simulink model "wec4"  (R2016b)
settings: Solver=ode4  StartTime=0  StopTime=1000  FixedStep=0.005  MaxStep=0.005  RelTol=1e-3  EnableMultiTasking=on
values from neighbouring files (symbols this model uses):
  arAdaptiveLawData = 1/2*zModelSimple.zModelPto.arFreq.*     zModelSimple.zModelPto.arMagnitude./     cos(zModelSimple.zModelPto.arPhase*pi/180+pi/2)    [IMPACT_Control.m]
  arAdaptiveLawDataX = 1/2*zModelSimpleX.zModelPto.arFreq.*         zModelSimpleX.zModelPto.arMagnitude./         cos(zModelSimpleX.zModelPto.arPhase*pi/180+pi/2)    [IMPACT_Control.m]
  arControllerRampGain = [0,0,1,1]    [IMPACT_Control.m]
  arControllerRampTime = [0 rStartRampTime rStartRampTime+rRampTimeLength 8000]    [IMPACT_Control.m]
  arEkfInitialisation = zeros(1,11)    [IMPACT_Control.m]
  arEkfInitialisationX = zeros(1,11)    [IMPACT_Control.m]
  arFrequency = zModelSimple.zModelPto.arFreq    [IMPACT_Control.m]
  arFrequencyRange = zModelSimple.zModelPto.arFreq    [IMPACT_Control.m]
  arFrequencyX = zModelSimpleX.zModelPto.arFreq    [IMPACT_Control.m]
  arImpedance = 1./zModelSimple.zModelPto.arMagnitude./zModelSimple.zModelPto.arFreq    [IMPACT_Control.m]
  arImpedanceX = 1./zModelSimpleX.zModelPto.arMagnitude./zModelSimpleX.zModelPto.arFreq    [IMPACT_Control.m]
  CentralPTOPreload = -1.6113e+07    (= -16113000)    [wecSimInputFile.m]
  F1 = [4.243 2.375 -12.243]    [wecSimInputFile.m]
  F2 = [4.243 -2.375 -12.243]    [wecSimInputFile.m]
  F3 = [-4.243 -2.375 -12.243]    [wecSimInputFile.m]
  F4 = [-4.243 2.375 -12.243]    [wecSimInputFile.m]
  FC = [0 0 -14]    [wecSimInputFile.m]
  iAdaptiveDamping = 0    [wec4IMPACT_Project.m]    (also in IMPACT_Control.m = handles.iAdaptiveDamping; wec1_IMPACT_Project.m; wec2_IMPACT_Project.m; wec3_IMPACT_Project.m)
  iControlType = 2    [wec4IMPACT_Project.m]    (also in IMPACT_Control.m = handles.iControlType; wec1_IMPACT_Project.m = 1; wec2_IMPACT_Project.m = 1; wec3_IMPACT_Project.m = 1)
  iPtoPositionConstraint = 1    [wec4IMPACT_Project.m]    (also in IMPACT_Control.m = handles.iPtoPositionConstraint; wec1_IMPACT_Project.m = 0; wec2_IMPACT_Project.m; wec3_IMPACT_Project.m)
  iSensorNoise = 0    [IMPACT_Control.m]
  m = m+1    (= 2)    [checkParamFile.m]
  PTOrotation = atan((T1(2)-F1(2))/(T1(1)-F1(1)))    [wecSimInputFile.m]
  rCogFloater = -8    [wec4_IMPACT_Model.m]    (also in paramInitial.m = get( handles.edit_rCogFloater, 'String' ); wec1_IMPACT_Model.m = -18; wec2_IMPACT_Model.m = -8.5; wec3_IMPACT_Model.m = -0.7)
  rCogSpar = -36.6    [wec4_IMPACT_Model.m]    (also in paramInitial.m = get( handles.edit_rCogSpar, 'String' ); wec3_IMPACT_Model.m = -21.3; wec3_IMPACT_Model2.m = -21.3)
  rDisplacementLimit = 10.000000    (= 10)    [wec4IMPACT_Project.m]    (also in IMPACT_Control.m = getValue(handles.edit_displacementLimit); wec1_IMPACT_Project.m; wec2_IMPACT_Project.m; wec3_IMPACT_Project.m = 3)
  rDisplacementLimitX = 10.000000    (= 10)    [wec4IMPACT_Project.m]    (also in IMPACT_Control.m = getValue(handles.edit_displacementLimitX); wec1_IMPACT_Project.m = 0; wec2_IMPACT_Project.m; wec3_IMPACT_Project.m = 0)
  rGainForAntiWIndUp = tfControllerDiscrete.rGain    [IMPACT_Control.m]
  rGainForAntiWIndUpX = tfControllerXDiscrete.rGain    [IMPACT_Control.m]
  rMaxForcePto = 300000000.000000    (= 300000000)    [wec4IMPACT_Project.m]    (also in IMPACT_Control.m = getValue(handles.edit_maxForcePto); wec1_IMPACT_Project.m = 1e+15; wec2_IMPACT_Project.m = 1e+15; wec3_IMPACT_Project.m = 1000000000)
  rMinForcePto = -300000000.000000    (= -300000000)    [wec4IMPACT_Project.m]    (also in IMPACT_Control.m = getValue(handles.edit_minForcePto); wec1_IMPACT_Project.m = -1e+15; wec2_IMPACT_Project.m = -1e+15; wec3_IMPACT_Project.m = -1000000000)
  rMooringX = 20000    [wec4_IMPACT_Model.m]    (also in paramInitial.m = get( handles.edit_rMooringX, 'String' ); wec3_IMPACT_Model.m = 10000; wec3_IMPACT_Model2.m = 10000)
  rMooringZ = 10000    [wec4_IMPACT_Model.m]    (also in paramInitial.m = get( handles.edit_rMooringZ, 'String' ); wec3_IMPACT_Model.m = 0; wec3_IMPACT_Model2.m = 0)
  rOutputSampleTime = 0.010000    (= 0.01)    [wec4IMPACT_Project.m]    (also in IMPACT_Control.m = getValue(handles.edit_outputSampleTime); wec1_IMPACT_Project.m; wec2_IMPACT_Project.m; wec3_IMPACT_Project.m)
  rPassiveDampingGain = -604830.000000    (= -604830)    [wec4IMPACT_Project.m]    (also in IMPACT_Control.m = getValue(handles.edit_gainPLD); wec1_IMPACT_Project.m = -214018.1537; wec2_IMPACT_Project.m = -1948070; wec3_IMPACT_Project.m = -519390)
  rPassiveDampingGainX = -278660.000000    (= -278660)    [wec4IMPACT_Project.m]    (also in IMPACT_Control.m = getValue(handles.edit_gainPLDX); wec1_IMPACT_Project.m = 0; wec2_IMPACT_Project.m = 0; wec3_IMPACT_Project.m = 0)
  rTetherPretension = 1.6113e+07    (= 16113000)    [wec4_IMPACT_Model.m]    (also in paramInitial.m = get( handles.edit_rTetherPretension, 'String' ); wec3_IMPACT_Model.m = 0; wec3_IMPACT_Model2.m = 0)
  rTetherSpring = 500000    [wec4_IMPACT_Model.m]    (also in paramInitial.m = get( handles.edit_rTetherSpring, 'String' ); wec3_IMPACT_Model.m = 0; wec3_IMPACT_Model2.m = 0)
  rUpperFrequencyLimit = EKFFloater.upperFreq    [IMPACT_Control.m]
  rXf = 4.243    [wec4AdditionalParams.m]
  rXs = 16.075    [wec4AdditionalParams.m]
  rYf = 2.375    [wec4AdditionalParams.m]
  rYs = 16.075    [wec4AdditionalParams.m]
  rZf = 4.243    [wec4AdditionalParams.m]
  rZs = 2.4350    (= 2.435)    [wec4AdditionalParams.m]
  rZTetherF = 6    [wec4AdditionalParams.m]
  rZTetherS = 2.4350    (= 2.435)    [wec4AdditionalParams.m]
  s = tf('s')    [wec4_IMPACT_Model.m]    (also in IMPACT_Control.m; wec1_IMPACT_Model.m; wec2_IMPACT_Model.m; wec3_IMPACT_Model.m)
  SidePTO1Preload = PreloadPTOCorner    (= 0)    [wecSimInputFile.m]
  SidePTO2Preload = PreloadPTOCorner    (= 0)    [wecSimInputFile.m]
  SidePTO3Preload = PreloadPTOCorner    (= 0)    [wecSimInputFile.m]
  SidePTO4Preload = PreloadPTOCorner    (= 0)    [wecSimInputFile.m]
  simu = simulationClass()    [wecSimInputFile.m]
  T1 = [16.075 16.075 -34.165]    [wecSimInputFile.m]
  T2 = [16.075 -16.075 -34.165]    [wecSimInputFile.m]
  T3 = [-16.075 -16.075 -34.165]    [wecSimInputFile.m]
  T4 = [-16.075 16.075 -34.165]    [wecSimInputFile.m]
  TC = [0 0 -34.165]    [wecSimInputFile.m]
  waves = waveClass('irregular')    [wecSimInputFile.m]
  Z = magPhaseToComplex(zModelTf)    [IMPACT_Control.m]
undefined symbols (not defined in the file or in its folder): arControllerDiscreteDen, arControllerDiscreteNum, arControllerDiscreteXDen, arControllerDiscreteXNum, arExcForceFloaterDen, arExcForceFloaterNum, arExcForceFloaterXDen, arExcForceFloaterXNum, arExcForceSparDen, arExcForceSparNum, arExcForceSparXDen, arExcForceSparXNum, arFexcFloaterDen, arFexcFloaterNum, arFexcFloaterXDen, arFexcFloaterXNum, arFexcSparDen, arFexcSparNum, arFexcSparXDen, arFexcSparXNum, Body, body, constraint, CTTime, deg, Elements, geometry, IRKB, kg, lenJ, mooring, N, pto, rAccelerationGainFloater, rAccelerationGainFloaterX, rAccelerationGainSpar, rAccelerationGainSparX, rad, rBuoyancyGainFloater, rBuoyancyGainFloaterX, rBuoyancyGainSpar, rBuoyancyGainSparX, rDampingGainFloater, rDampingGainFloaterX, rDampingGainSpar, rDampingGainSparX, Rigid, rMaxFocePto, wec4_float, wec4_reactor, WECSim_Lib, X, Y
libraries: nesl_utility x380, sm_lib x170, vrlib x91, simulink x12, WECSim_Lib x4
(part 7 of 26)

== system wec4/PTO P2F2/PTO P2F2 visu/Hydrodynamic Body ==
  Additional Linear Damping Force Calculation : Subsystem
  B2B Subsystem : Subsystem  Variant=on
  Bus Creator : BusCreator  Inputs=6
  Bus Creator1 : BusCreator  Inputs=3
  Bus Selector1 : BusSelector  OutputSignals=F_Excitation,F_RadiationDamping,F_AddedMass,F_Restoring,F_MorrisonAndViscous,F_LinearDamping
  Bus Selector2 : BusSelector  OutputSignals=disp,vel,acc
  Hydrostatic Restoring Force Calculation : Subsystem
  Morrison Element and ViscousDampingForceCalculation : Subsystem
  Nonlinear Wave Elevation : Subsystem  TreatAsAtomicUnit=on  SystemSampleTime=simu.dtNL
  Structure : Subsystem
  Sum : Sum  Inputs=+-----
  To Workspace : ToWorkspace  VariableName=body5_out  SaveFormat=Structure With Time  SampleTime=-1
  Wave Diffraction and Excitation Force Calculation : Subsystem
  Wave Radiation Forces Calculation : Subsystem
  Conn : PMIOPort  Port=1  Side=Right
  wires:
  Additional Linear Damping Force Calculation/1(F_LinearDamping) -> Bus Creator/6
  Bus Creator/1 -> Bus Selector1/1, Bus Creator1/3  "BUS(7): Forces"
  Bus Selector2/1 -> [disp5]  "<disp>"
  Bus Selector2/3 -> [acc5]  "<acc>"
  Bus Selector2/2 -> [vel5]  "<vel>"
  Structure/1(Response) -> Bus Creator1/1, Bus Selector2/1
  Sum/1 -> Bus Creator1/2, Structure/1(Total Force)  "F_Total"
  Bus Creator1/1 -> To Workspace/1
  Bus Selector1/4 -> Sum/4  "<F_Restoring>"
  Bus Selector1/3 -> Sum/3  "<F_AddedMass>"
  Bus Selector1/5 -> Sum/5  "<F_MorrisonAndViscous>"
  Bus Selector1/2 -> Sum/2  "<F_RadiationDamping>"
  Bus Selector1/1 -> Sum/1  "<F_Excitation>"
  Bus Selector1/6 -> Sum/6  "<F_LinearDamping>"
  [acc5] -> B2B Subsystem/2(acc_in), Morrison Element and ViscousDampingForceCalculation/2(Acceleration)
  [vel5] -> Morrison Element and ViscousDampingForceCalculation/3(Velocity), Additional Linear Damping Force Calculation/1(Velocity), B2B Subsystem/1(vel_in)
  B2B Subsystem/2(acc) -> Wave Radiation Forces Calculation/2(Acceleration)
  B2B Subsystem/1(vel) -> Wave Radiation Forces Calculation/1(Velocity)
  [disp5] -> Hydrostatic Restoring Force Calculation/1(Displacement), Morrison Element and ViscousDampingForceCalculation/1(Displacement), Nonlinear Wave Elevation/1(Displacement), Wave Diffraction and Excitation Force Calculation/2(Displacement)
  Nonlinear Wave Elevation/1(Wave Elevation) -> Wave Diffraction and Excitation Force Calculation/3(WaveElv), Hydrostatic Restoring Force Calculation/2(Wave Elv)
  Hydrostatic Restoring Force Calculation/1(F_Restoring) -> Bus Creator/4
  Wave Radiation Forces Calculation/1(F_RadiationDamping) -> Bus Creator/2
  Wave Diffraction and Excitation Force Calculation/1(F_Excitation) -> Bus Creator/1
  Wave Radiation Forces Calculation/2(F_AddedMass) -> Bus Creator/3
  [Clock] -> Nonlinear Wave Elevation/2(Time), Wave Diffraction and Excitation Force Calculation/1(Time), Morrison Element and ViscousDampingForceCalculation/4(Time), Wave Radiation Forces Calculation/3(Time)
  Morrison Element and ViscousDampingForceCalculation/1(F_MorrisonAndViscous) -> Bus Creator/5
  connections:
  Conn/RConn1 -- Structure/RConn1

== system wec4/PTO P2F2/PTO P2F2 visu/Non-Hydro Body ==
  Bus Creator : BusCreator  Inputs=6
  Bus Creator1 : BusCreator  Inputs=3
  Bus Selector1 : BusSelector  OutputSignals=F_Excitation,F_RadiationDamping,F_AddedMass,F_Restoring,F_MorrisonAndViscous,F_LinearDamping
  Constant{,1..3,5} (5 alike) : Constant  Value=[0 0 0 0 0 0]
  Structure : Subsystem
  Sum : Sum  Inputs=+-----
  To Workspace : ToWorkspace  VariableName=body5_out  SaveFormat=Structure With Time  SampleTime=-1
  Weight and Buoyancy : Subsystem
  Conn : PMIOPort  Port=1  Side=Right
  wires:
  Bus Creator/1 -> Bus Creator1/3, Bus Selector1/1  "BUS(7): Forces"
  Structure/1(Response) -> Bus Creator1/1
  Sum/1 -> Bus Creator1/2, Structure/1(Total Force)  "F_Total"
  Bus Creator1/1 -> To Workspace/1
  Bus Selector1/4 -> Sum/4  "<F_Restoring>"
  Bus Selector1/3 -> Sum/3  "<F_AddedMass>"
  Bus Selector1/5 -> Sum/5  "<F_MorrisonAndViscous>"
  Bus Selector1/2 -> Sum/2  "<F_RadiationDamping>"
  Bus Selector1/1 -> Sum/1  "<F_Excitation>"
  Bus Selector1/6 -> Sum/6  "<F_LinearDamping>"
  Constant5/1 -> Bus Creator/6  "F_LinearDamping"
  Constant3/1 -> Bus Creator/5  "F_MorrisonAndViscous"
  Constant2/1 -> Bus Creator/3  "F_AddedMass"
  Constant1/1 -> Bus Creator/2  "F_RadiationDamping"
  Constant/1 -> Bus Creator/1  "F_Excitation"
  Weight and Buoyancy/1(Out1) -> Bus Creator/4  "F_Restoring"
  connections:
  Conn/RConn1 -- Structure/RConn1

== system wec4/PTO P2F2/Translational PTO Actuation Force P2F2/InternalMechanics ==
  note: Calculate PTO force and power. F_pto = k*x + c*v, where F_pto is the force the PTO applies to the body (at the PTO location), x and v are the joint position and velocity. The power extracted is P = c * v^2
  Position : Inport
  Velocity : Inport  Port=2
  Add : Sum  Inputs=--
  Math Function : Math  Operator=square
  PCC Damping Coefficient : Constant  Value=pto.c
  PCC Stiffness Coefficient : Constant  Value=pto.k
  Product : Product  Inputs=**
  Product1 : Product  Inputs=**
  Product2 : Product  Inputs=**
  Force : Outport
  Power : Outport  Port=2
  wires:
  PCC Damping Coefficient/1 -> Product2/1, Product1/1
  Product2/1 -> Power/1
  Velocity/1 -> Math Function/1, Product1/2
  PCC Stiffness Coefficient/1 -> Product/2
  Position/1 -> Product/1
  Add/1 -> Force/1
  Math Function/1 -> Product2/2
  Product/1 -> Add/1
  Product1/1 -> Add/2

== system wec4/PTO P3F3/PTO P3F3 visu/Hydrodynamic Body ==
  Additional Linear Damping Force Calculation : Subsystem
  B2B Subsystem : Subsystem  Variant=on
  Bus Creator : BusCreator  Inputs=6
  Bus Creator1 : BusCreator  Inputs=3
  Bus Selector1 : BusSelector  OutputSignals=F_Excitation,F_RadiationDamping,F_AddedMass,F_Restoring,F_MorrisonAndViscous,F_LinearDamping
  Bus Selector2 : BusSelector  OutputSignals=disp,vel,acc
  Hydrostatic Restoring Force Calculation : Subsystem
  Morrison Element and ViscousDampingForceCalculation : Subsystem
  Nonlinear Wave Elevation : Subsystem  TreatAsAtomicUnit=on  SystemSampleTime=simu.dtNL
  Structure : Subsystem
  Sum : Sum  Inputs=+-----
  To Workspace : ToWorkspace  VariableName=body6_out  SaveFormat=Structure With Time  SampleTime=-1
  Wave Diffraction and Excitation Force Calculation : Subsystem
  Wave Radiation Forces Calculation : Subsystem
  Conn : PMIOPort  Port=1  Side=Right
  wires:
  Additional Linear Damping Force Calculation/1(F_LinearDamping) -> Bus Creator/6
  Bus Creator/1 -> Bus Selector1/1, Bus Creator1/3  "BUS(7): Forces"
  Bus Selector2/1 -> [disp6]  "<disp>"
  Bus Selector2/3 -> [acc6]  "<acc>"
  Bus Selector2/2 -> [vel6]  "<vel>"
  Structure/1(Response) -> Bus Creator1/1, Bus Selector2/1
  Sum/1 -> Bus Creator1/2, Structure/1(Total Force)  "F_Total"
  Bus Creator1/1 -> To Workspace/1
  Bus Selector1/4 -> Sum/4  "<F_Restoring>"
  Bus Selector1/3 -> Sum/3  "<F_AddedMass>"
  Bus Selector1/5 -> Sum/5  "<F_MorrisonAndViscous>"
  Bus Selector1/2 -> Sum/2  "<F_RadiationDamping>"
  Bus Selector1/1 -> Sum/1  "<F_Excitation>"
  Bus Selector1/6 -> Sum/6  "<F_LinearDamping>"
  [acc6] -> B2B Subsystem/2(acc_in), Morrison Element and ViscousDampingForceCalculation/2(Acceleration)
  [vel6] -> Morrison Element and ViscousDampingForceCalculation/3(Velocity), Additional Linear Damping Force Calculation/1(Velocity), B2B Subsystem/1(vel_in)
  B2B Subsystem/2(acc) -> Wave Radiation Forces Calculation/2(Acceleration)
  B2B Subsystem/1(vel) -> Wave Radiation Forces Calculation/1(Velocity)
  [disp6] -> Hydrostatic Restoring Force Calculation/1(Displacement), Morrison Element and ViscousDampingForceCalculation/1(Displacement), Nonlinear Wave Elevation/1(Displacement), Wave Diffraction and Excitation Force Calculation/2(Displacement)
  Nonlinear Wave Elevation/1(Wave Elevation) -> Wave Diffraction and Excitation Force Calculation/3(WaveElv), Hydrostatic Restoring Force Calculation/2(Wave Elv)
  Hydrostatic Restoring Force Calculation/1(F_Restoring) -> Bus Creator/4
  Wave Radiation Forces Calculation/1(F_RadiationDamping) -> Bus Creator/2
  Wave Diffraction and Excitation Force Calculation/1(F_Excitation) -> Bus Creator/1
  Wave Radiation Forces Calculation/2(F_AddedMass) -> Bus Creator/3
  [Clock] -> Nonlinear Wave Elevation/2(Time), Wave Diffraction and Excitation Force Calculation/1(Time), Morrison Element and ViscousDampingForceCalculation/4(Time), Wave Radiation Forces Calculation/3(Time)
  Morrison Element and ViscousDampingForceCalculation/1(F_MorrisonAndViscous) -> Bus Creator/5
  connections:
  Conn/RConn1 -- Structure/RConn1

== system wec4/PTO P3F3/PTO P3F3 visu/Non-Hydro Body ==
  Bus Creator : BusCreator  Inputs=6
  Bus Creator1 : BusCreator  Inputs=3
  Bus Selector1 : BusSelector  OutputSignals=F_Excitation,F_RadiationDamping,F_AddedMass,F_Restoring,F_MorrisonAndViscous,F_LinearDamping
  Constant{,1..3,5} (5 alike) : Constant  Value=[0 0 0 0 0 0]
  Structure : Subsystem
  Sum : Sum  Inputs=+-----
  To Workspace : ToWorkspace  VariableName=body6_out  SaveFormat=Structure With Time  SampleTime=-1
  Weight and Buoyancy : Subsystem
  Conn : PMIOPort  Port=1  Side=Right
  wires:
  Bus Creator/1 -> Bus Creator1/3, Bus Selector1/1  "BUS(7): Forces"
  Structure/1(Response) -> Bus Creator1/1
  Sum/1 -> Bus Creator1/2, Structure/1(Total Force)  "F_Total"
  Bus Creator1/1 -> To Workspace/1
  Bus Selector1/4 -> Sum/4  "<F_Restoring>"
  Bus Selector1/3 -> Sum/3  "<F_AddedMass>"
  Bus Selector1/5 -> Sum/5  "<F_MorrisonAndViscous>"
  Bus Selector1/2 -> Sum/2  "<F_RadiationDamping>"
  Bus Selector1/1 -> Sum/1  "<F_Excitation>"
  Bus Selector1/6 -> Sum/6  "<F_LinearDamping>"
  Constant5/1 -> Bus Creator/6  "F_LinearDamping"
  Constant3/1 -> Bus Creator/5  "F_MorrisonAndViscous"
  Constant2/1 -> Bus Creator/3  "F_AddedMass"
  Constant1/1 -> Bus Creator/2  "F_RadiationDamping"
  Constant/1 -> Bus Creator/1  "F_Excitation"
  Weight and Buoyancy/1(Out1) -> Bus Creator/4  "F_Restoring"
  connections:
  Conn/RConn1 -- Structure/RConn1

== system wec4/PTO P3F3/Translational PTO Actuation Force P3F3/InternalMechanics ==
  note: Calculate PTO force and power. F_pto = k*x + c*v, where F_pto is the force the PTO applies to the body (at the PTO location), x and v are the joint position and velocity. The power extracted is P = c * v^2
  Position : Inport
  Velocity : Inport  Port=2
  Add : Sum  Inputs=--
  Math Function : Math  Operator=square
  PCC Damping Coefficient : Constant  Value=pto.c
  PCC Stiffness Coefficient : Constant  Value=pto.k
  Product : Product  Inputs=**
  Product1 : Product  Inputs=**
  Product2 : Product  Inputs=**
  Force : Outport
  Power : Outport  Port=2
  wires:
  PCC Damping Coefficient/1 -> Product2/1, Product1/1
  Product2/1 -> Power/1
  Velocity/1 -> Math Function/1, Product1/2
  PCC Stiffness Coefficient/1 -> Product/2
  Position/1 -> Product/1
  Add/1 -> Force/1
  Math Function/1 -> Product2/2
  Product/1 -> Add/1
  Product1/1 -> Add/2

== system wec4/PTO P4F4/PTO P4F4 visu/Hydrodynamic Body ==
  Additional Linear Damping Force Calculation : Subsystem
  B2B Subsystem : Subsystem  Variant=on
  Bus Creator : BusCreator  Inputs=6
  Bus Creator1 : BusCreator  Inputs=3
  Bus Selector1 : BusSelector  OutputSignals=F_Excitation,F_RadiationDamping,F_AddedMass,F_Restoring,F_MorrisonAndViscous,F_LinearDamping
  Bus Selector2 : BusSelector  OutputSignals=disp,vel,acc
  Hydrostatic Restoring Force Calculation : Subsystem
  Morrison Element and ViscousDampingForceCalculation : Subsystem
  Nonlinear Wave Elevation : Subsystem  TreatAsAtomicUnit=on  SystemSampleTime=simu.dtNL
  Structure : Subsystem
  Sum : Sum  Inputs=+-----
  To Workspace : ToWorkspace  VariableName=body7_out  SaveFormat=Structure With Time  SampleTime=-1
  Wave Diffraction and Excitation Force Calculation : Subsystem
  Wave Radiation Forces Calculation : Subsystem
  Conn : PMIOPort  Port=1  Side=Right
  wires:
  Additional Linear Damping Force Calculation/1(F_LinearDamping) -> Bus Creator/6
  Bus Creator/1 -> Bus Selector1/1, Bus Creator1/3  "BUS(7): Forces"
  Bus Selector2/1 -> [disp7]  "<disp>"
  Bus Selector2/3 -> [acc7]  "<acc>"
  Bus Selector2/2 -> [vel7]  "<vel>"
  Structure/1(Response) -> Bus Creator1/1, Bus Selector2/1
  Sum/1 -> Bus Creator1/2, Structure/1(Total Force)  "F_Total"
  Bus Creator1/1 -> To Workspace/1
  Bus Selector1/4 -> Sum/4  "<F_Restoring>"
  Bus Selector1/3 -> Sum/3  "<F_AddedMass>"
  Bus Selector1/5 -> Sum/5  "<F_MorrisonAndViscous>"
  Bus Selector1/2 -> Sum/2  "<F_RadiationDamping>"
  Bus Selector1/1 -> Sum/1  "<F_Excitation>"
  Bus Selector1/6 -> Sum/6  "<F_LinearDamping>"
  [acc7] -> B2B Subsystem/2(acc_in), Morrison Element and ViscousDampingForceCalculation/2(Acceleration)
  [vel7] -> Morrison Element and ViscousDampingForceCalculation/3(Velocity), Additional Linear Damping Force Calculation/1(Velocity), B2B Subsystem/1(vel_in)
  B2B Subsystem/2(acc) -> Wave Radiation Forces Calculation/2(Acceleration)
  B2B Subsystem/1(vel) -> Wave Radiation Forces Calculation/1(Velocity)
  [disp7] -> Hydrostatic Restoring Force Calculation/1(Displacement), Morrison Element and ViscousDampingForceCalculation/1(Displacement), Nonlinear Wave Elevation/1(Displacement), Wave Diffraction and Excitation Force Calculation/2(Displacement)
  Nonlinear Wave Elevation/1(Wave Elevation) -> Wave Diffraction and Excitation Force Calculation/3(WaveElv), Hydrostatic Restoring Force Calculation/2(Wave Elv)
  Hydrostatic Restoring Force Calculation/1(F_Restoring) -> Bus Creator/4
  Wave Radiation Forces Calculation/1(F_RadiationDamping) -> Bus Creator/2
  Wave Diffraction and Excitation Force Calculation/1(F_Excitation) -> Bus Creator/1
  Wave Radiation Forces Calculation/2(F_AddedMass) -> Bus Creator/3
  [Clock] -> Nonlinear Wave Elevation/2(Time), Wave Diffraction and Excitation Force Calculation/1(Time), Morrison Element and ViscousDampingForceCalculation/4(Time), Wave Radiation Forces Calculation/3(Time)
  Morrison Element and ViscousDampingForceCalculation/1(F_MorrisonAndViscous) -> Bus Creator/5
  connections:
  Conn/RConn1 -- Structure/RConn1

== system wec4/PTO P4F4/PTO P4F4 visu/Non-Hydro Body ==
  Bus Creator : BusCreator  Inputs=6
  Bus Creator1 : BusCreator  Inputs=3
  Bus Selector1 : BusSelector  OutputSignals=F_Excitation,F_RadiationDamping,F_AddedMass,F_Restoring,F_MorrisonAndViscous,F_LinearDamping
  Constant{,1..3,5} (5 alike) : Constant  Value=[0 0 0 0 0 0]
  Structure : Subsystem
  Sum : Sum  Inputs=+-----
  To Workspace : ToWorkspace  VariableName=body7_out  SaveFormat=Structure With Time  SampleTime=-1
  Weight and Buoyancy : Subsystem
  Conn : PMIOPort  Port=1  Side=Right
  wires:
  Bus Creator/1 -> Bus Creator1/3, Bus Selector1/1  "BUS(7): Forces"
  Structure/1(Response) -> Bus Creator1/1
  Sum/1 -> Bus Creator1/2, Structure/1(Total Force)  "F_Total"
  Bus Creator1/1 -> To Workspace/1
  Bus Selector1/4 -> Sum/4  "<F_Restoring>"
  Bus Selector1/3 -> Sum/3  "<F_AddedMass>"
  Bus Selector1/5 -> Sum/5  "<F_MorrisonAndViscous>"
  Bus Selector1/2 -> Sum/2  "<F_RadiationDamping>"
  Bus Selector1/1 -> Sum/1  "<F_Excitation>"
  Bus Selector1/6 -> Sum/6  "<F_LinearDamping>"
  Constant5/1 -> Bus Creator/6  "F_LinearDamping"
  Constant3/1 -> Bus Creator/5  "F_MorrisonAndViscous"
  Constant2/1 -> Bus Creator/3  "F_AddedMass"
  Constant1/1 -> Bus Creator/2  "F_RadiationDamping"
  Constant/1 -> Bus Creator/1  "F_Excitation"
  Weight and Buoyancy/1(Out1) -> Bus Creator/4  "F_Restoring"
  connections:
  Conn/RConn1 -- Structure/RConn1

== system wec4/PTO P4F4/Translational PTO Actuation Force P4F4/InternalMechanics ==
  note: Calculate PTO force and power. F_pto = k*x + c*v, where F_pto is the force the PTO applies to the body (at the PTO location), x and v are the joint position and velocity. The power extracted is P = c * v^2
  Position : Inport
  Velocity : Inport  Port=2
  Add : Sum  Inputs=--
  Math Function : Math  Operator=square
  PCC Damping Coefficient : Constant  Value=pto.c
  PCC Stiffness Coefficient : Constant  Value=pto.k
  Product : Product  Inputs=**
  Product1 : Product  Inputs=**
  Product2 : Product  Inputs=**
  Force : Outport
  Power : Outport  Port=2
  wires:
  PCC Damping Coefficient/1 -> Product2/1, Product1/1
  Product2/1 -> Power/1
  Velocity/1 -> Math Function/1, Product1/2
  PCC Stiffness Coefficient/1 -> Product/2
  Position/1 -> Product/1
  Add/1 -> Force/1
  Math Function/1 -> Product2/2
  Product/1 -> Add/1
  Product1/1 -> Add/2

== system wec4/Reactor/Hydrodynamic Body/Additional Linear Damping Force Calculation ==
  Velocity : Inport
  Additional Linear Damping Matrix (diagonal) : Constant  Value=body.hydroForce.linearDamping
  Product1 : Product  Multiplication=Matrix(*)
  F_LinearDamping : Outport
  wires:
  Velocity/1 -> Product1/2  "v"
  Product1/1 -> F_LinearDamping/1  "F_LinearDamping"
  Additional Linear Damping Matrix (diagonal)/1 -> Product1/1  "C"

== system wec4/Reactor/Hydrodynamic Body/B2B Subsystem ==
  note: 1) Add Subsystem or Model blocks as valid variant choices. 2) You cannot connect blocks at this level. At simulation, connectivity is automatically determined, based on the active variant and port name matching.
  vel_in : Inport
  acc_in : Inport  Port=2
  B2B : Subsystem  VariantControl=sv_B2B
  noB2B : Subsystem  VariantControl=sv_noB2B
  vel : Outport
  acc : Outport  Port=2

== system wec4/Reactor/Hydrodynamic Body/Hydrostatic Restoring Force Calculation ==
  Displacement : Inport
  Wave Elv : Inport  Port=2
  Add : Sum  Inputs=+-
  Center of Gravity : Constant  Value=body.cg
  Constant : Constant  Value=[0 0 0]
  Linear and Nonlinear Restoring Force Variant Subsystem : Subsystem  Variant=on
  Mux : Mux  Inputs=2
  F_Restoring : Outport
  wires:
  Add/1 -> Linear and Nonlinear Restoring Force Variant Subsystem/1(In1)  "x_cg"
  Wave Elv/1 -> Linear and Nonlinear Restoring Force Variant Subsystem/2(In2)
  Constant/1 -> Mux/2
  Center of Gravity/1 -> Mux/1  "cg"
  Mux/1 -> Add/2
  Linear and Nonlinear Restoring Force Variant Subsystem/1(Out1) -> F_Restoring/1  "F_Restoring"
  Displacement/1 -> Add/1  "x"

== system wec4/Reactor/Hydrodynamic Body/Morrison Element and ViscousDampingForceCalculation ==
  Displacement : Inport
  Acceleration : Inport  Port=2
  Velocity : Inport  Port=3
  Time : Inport  Port=4
  Abs1 : Abs
  Morrison Element Variant Subsystem : Subsystem  Variant=on
  Product : Product
  Product1 : Product  Multiplication=Matrix(*)
  Transport Delay : TransportDelay  DelayTime=10e-8
  "VisSum " : Sum  Inputs=+-
  "Viscous Damping Matrix (diagonal) " : Constant  Value=body.hydroForce.visDrag
  F_MorrisonAndViscous : Outport
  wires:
  Time/1 -> Morrison Element Variant Subsystem/4(time)
  Morrison Element Variant Subsystem/1(morison_force) -> "VisSum "/2
  Displacement/1 -> Morrison Element Variant Subsystem/1(displacement)
  Product/1 -> Product1/2  "v * |v|"
  "Viscous Damping Matrix (diagonal) "/1 -> Product1/1  "0.5 * cd * rho *A"
  Product1/1 -> "VisSum "/1
  Abs1/1 -> Product/2
  Acceleration/1 -> Transport Delay/1
  Transport Delay/1 -> Morrison Element Variant Subsystem/3(acceleration)
  "VisSum "/1 -> F_MorrisonAndViscous/1  "F_MorrisonAndViscous"
  Velocity/1 -> Abs1/1, Product/1, Morrison Element Variant Subsystem/2(velocity)

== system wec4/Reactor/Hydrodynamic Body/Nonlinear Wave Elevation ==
  Displacement : Inport
  Time : Inport  Port=2
  Add : Sum  Inputs=+-
  Center of Gravity : Constant  Value=body.cg
  Constant : Constant  Value=[0 0 0]
  Linear or Instantaneous Free Surface : Subsystem  Variant=on
  Mux : Mux  Inputs=2
  Wave Elevation : Outport
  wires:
  Time/1 -> Linear or Instantaneous Free Surface/2(In2)
  Constant/1 -> Mux/2
  Center of Gravity/1 -> Mux/1  "cg"
  Mux/1 -> Add/2
  Add/1 -> Linear or Instantaneous Free Surface/1(In1)  "x_cg"
  Linear or Instantaneous Free Surface/1(Out1) -> Wave Elevation/1
  Displacement/1 -> Add/1  "x"

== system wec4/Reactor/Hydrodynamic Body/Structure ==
  Total Force : Inport
  Body Properties : sm_lib/Body Elements/Solid  InertiaType=Custom  Mass=body.mass  MassUnits=kg  CenterOfMass=[0 0 0]  CenterOfMassUnits=m  MomentsOfInertia=body.momOfInertia  MomentsOfInertiaUnits=kg*m^2  ProductsOfInertia=[0 0 0]  ProductsOfInertiaUnits=kg*m^2  DensityBased=on  Density=1000  DensityUnits=kg/(m^3)  DoExposeReferenceFrame=on  SerializedFrames=<Frames/>  GraphicType=FromGeometry  MarkerShape=Sphere  MarkerSize=10  MarkerSizeUnits=m  GraphicVisPropType=SimpleVisualProperties  GraphicDiffuseColor=body.viz.color  GraphicSpecularColor=[0.5 0.5 0.5 1.0]  GraphicAmbientColor=[0.15 0.15 0.15 1.0]  GraphicEmissiveColor=[0.0 0.0 0.0 1.0]  GraphicShininess=75  GraphicOpacity=body.viz.opacity  GeometryShape=FromFile  RectangleSize=[1 1]  RectangleSizeUnits=m  BrickDimensions=[1 1 1]  BrickDimensionUnits=m  CylinderRadius=1  CylinderRadiusUnits=m  CylinderLength=1  CylinderLengthUnits=m  SphereRadius=1  SphereRadiusUnits=m  EllipsoidRadii=[1 1 1]  EllipsoidRadiiUnits=m  ExtrusionCrossSection=[1 1; -1 1; -1 -1; 1 -1]  ExtrusionCrossSectionUnits=m  ExtrusionLength=1  ExtrusionLengthUnits=m  PolygonNumSides=3  PolygonOuterRadius=1  PolygonOuterRadiusUnits=m  ExtGeomFileType=STL  ExtGeomFileName=.\geometry\wec4_reactor.stl  ExtGeomFileUnits=m  RevolutionCrossSection=[1 1; 1 -1; 2 -1; 2 1]  RevolutionCrossSectionUnits=m  RevolutionExtent=Full  RevolutionAngle=180  RevolutionAngleUnits=deg
  External Force and Torque : sm_lib/Forces and Torques/External Force and Torque  ForceResolutionFrame=World  EnableForceX=off  EnableForceY=off  EnableForceZ=off  EnableForce=on  TorqueResolutionFrame=World  EnableTorqueX=off  EnableTorqueY=off  EnableTorqueZ=off  EnableTorque=on
  Motion Sensor : Subsystem
  Rigid Transform (Setup CG) : sm_lib/Frames and Transforms/Rigid Transform  TranslationMethod=Cartesian  TranslationStandardOffset=0  TranslationLengthUnit=m  TranslationStandardAxis=+Z  TranslationCartesianOffset=body.cg  TranslationROffset=0  TranslationROffsetUnits=m  TranslationZOffset=0  TranslationZOffsetUnits=m  TranslationThetaOffset=0  TranslationThetaOffsetUnits=deg  RotationMethod=None  RotationAngleUnits=rad  RotationStandardAxis=+Y  RotationAngle=0.05  RotationArbitraryAxis=[0.57735026918962584 0.57735026918962584 0.57735026918962584]  FollAlignAxisA=+X  BaseAlignAxisA=+Y  FollAlignAxisB=+Y  BaseAlignAxisB=+Z  RotationSequenceAxes=FollowerAxes  RotationSequence=XYX  RotationSequenceAngles=[0 0 0]  RotationSequenceAnglesUnits=deg  RotationMatrix=[1 0 0; 0 1 0; 0 0 1]
  Rigid Transform (Setup Initial Disp) : sm_lib/Frames and Transforms/Rigid Transform  TranslationMethod=Cartesian  TranslationStandardOffset=0  TranslationLengthUnit=m  TranslationStandardAxis=+Z  TranslationCartesianOffset=body.initDisp.initLinDisp  TranslationROffset=0  TranslationROffsetUnits=m  TranslationZOffset=0  TranslationZOffsetUnits=m  TranslationThetaOffset=0  TranslationThetaOffsetUnits=deg  RotationMethod=ArbitraryAxis  RotationAngleUnits=rad  RotationStandardAxis=+Y  RotationAngle=body.initDisp.initAngularDispAngle  RotationArbitraryAxis=body.initDisp.initAngularDispAxis  FollAlignAxisA=+X  BaseAlignAxisA=+Y  FollAlignAxisB=+Y  BaseAlignAxisB=+Z  RotationSequenceAxes=FollowerAxes  RotationSequence=XYX  RotationSequenceAngles=[0 0 0]  RotationSequenceAnglesUnits=deg  RotationMatrix=[1 0 0; 0 1 0; 0 0 1]
  Selector : Selector  InputPortWidth=6  IndexOptions=Index vector (dialog)  Indices=[1:3]  OutputSizes=1
  Selector1 : Selector  InputPortWidth=6  IndexOptions=Index vector (dialog)  Indices=[4:6]  OutputSizes=1
  Simulink-PS Converter1 : nesl_utility/Simulink-PS Converter  PhysicalDomain=network_engine_domain  SubClassName=ps_input  LeftPortType=input  RightPortType=output  PseudoPeriodic=off  Frequencies=[]  NoiseDistribution=none  NoiseParameters=[]  Unit=1  AffineConversion=off  InputFiltering=off  SimscapeFilterOrder=1  InputFilterTimeConstant=0.001  UdotUserProvided=1
  Simulink-PS Converter2 : nesl_utility/Simulink-PS Converter  PhysicalDomain=network_engine_domain  SubClassName=ps_input  LeftPortType=input  RightPortType=output  PseudoPeriodic=off  Frequencies=[]  NoiseDistribution=none  NoiseParameters=[]  Unit=1  AffineConversion=off  InputFiltering=off  SimscapeFilterOrder=1  InputFilterTimeConstant=0.001  UdotUserProvided=1
  World Frame : sm_lib/Frames and Transforms/World Frame
  Conn Free Surface : PMIOPort  Port=1  Side=Right
  Response : Outport
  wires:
  Total Force/1 -> Selector1/1, Selector/1
  Selector/1 -> Simulink-PS Converter1/1
  Selector1/1 -> Simulink-PS Converter2/1
  Motion Sensor/1(Response) -> Response/1
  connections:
  External Force and Torque/LConn1 -- Simulink-PS Converter1/RConn1
  External Force and Torque/LConn2 -- Simulink-PS Converter2/RConn1
  Rigid Transform (Setup Initial Disp)/RConn1 -- Body Properties/RConn1 -- External Force and Torque/RConn1 -- Motion Sensor/RConn1
  Conn Free Surface/RConn1 -- Rigid Transform (Setup CG)/LConn1
  Rigid Transform (Setup Initial Disp)/LConn1 -- Rigid Transform (Setup CG)/RConn1
  World Frame/RConn1 -- Motion Sensor/LConn1

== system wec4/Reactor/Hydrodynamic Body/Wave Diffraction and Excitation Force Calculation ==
  Time : Inport
  Displacement : Inport  Port=2
  WaveElv : Inport  Port=3
  Add : Sum
  If2 : If  NumInputs=2  IfExpression=u1 < u2
  Linear Wave Excitation Force Variant Subsystem : Subsystem  Variant=on
  Merge1 : Merge
  No Ramp Function : Subsystem  TreatAsAtomicUnit=on
  Nonlinear FK Force Variant Subsystem : Subsystem  Variant=on
  Product : Product
  Ramp Function : Subsystem  TreatAsAtomicUnit=on
  Ramp Function Time : Constant  Value=simu.rampTime
  F_Excitation : Outport  PortDimensions=6
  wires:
  Nonlinear FK Force Variant Subsystem/1(Out1) -> Add/2
  Linear Wave Excitation Force Variant Subsystem/1(Out1) -> Add/1
  WaveElv/1 -> Nonlinear FK Force Variant Subsystem/3(In3)
  Displacement/1 -> Nonlinear FK Force Variant Subsystem/2(In2)
  Product/1 -> F_Excitation/1  "F_Excitation"
  Add/1 -> Product/2  "F_wave"
  Time/1 -> If2/1, Ramp Function/1(Time), Nonlinear FK Force Variant Subsystem/1(In1), Linear Wave Excitation Force Variant Subsystem/1(In1)
  Merge1/1 -> Product/1  "R"
  Ramp Function Time/1 -> If2/2
  If2/2 -> No Ramp Function/Action
  If2/1 -> Ramp Function/Action
  Ramp Function/1(R) -> Merge1/1
  No Ramp Function/1(R) -> Merge1/2

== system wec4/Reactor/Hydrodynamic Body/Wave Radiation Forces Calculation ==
  Velocity : Inport
  Acceleration : Inport  Port=2
  Time : Inport  Port=3
  Added Mass Matrix : Constant  Value=body.hydroForce.fAddedMass
  Product1 : Product  Multiplication=Matrix(*)
  SS CI and Constant-Damping-CoeVariant Subsystem : Subsystem  Variant=on
  Transport Delay : TransportDelay  DelayTime=10e-8
  F_RadiationDamping : Outport
  F_AddedMass : Outport  Port=2
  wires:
  Time/1 -> SS CI and Constant-Damping-CoeVariant Subsystem/2(In2)
  Acceleration/1 -> Transport Delay/1
  Transport Delay/1 -> Product1/2
  SS CI and Constant-Damping-CoeVariant Subsystem/1(Out1) -> F_RadiationDamping/1  "F_RadiationDamping"
  Velocity/1 -> SS CI and Constant-Damping-CoeVariant Subsystem/1(In1)
  Product1/1 -> F_AddedMass/1  "F_AddedMass"
  Added Mass Matrix/1 -> Product1/1

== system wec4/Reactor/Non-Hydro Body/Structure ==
  Total Force : Inport
  Body Properties : sm_lib/Body Elements/Solid  InertiaType=Custom  Mass=body.mass  MassUnits=kg  CenterOfMass=[0 0 0]  CenterOfMassUnits=m  MomentsOfInertia=body.momOfInertia  MomentsOfInertiaUnits=kg*m^2  ProductsOfInertia=[0 0 0]  ProductsOfInertiaUnits=kg*m^2  DensityBased=on  Density=1000  DensityUnits=kg/(m^3)  DoExposeReferenceFrame=on  SerializedFrames=<Frames/>  GraphicType=FromGeometry  MarkerShape=Sphere  MarkerSize=10  MarkerSizeUnits=m  GraphicVisPropType=SimpleVisualProperties  GraphicDiffuseColor=body.viz.color  GraphicSpecularColor=[0.5 0.5 0.5 1.0]  GraphicAmbientColor=[0.15 0.15 0.15 1.0]  GraphicEmissiveColor=[0.0 0.0 0.0 1.0]  GraphicShininess=75  GraphicOpacity=body.viz.opacity  GeometryShape=FromFile  RectangleSize=[1 1]  RectangleSizeUnits=m  BrickDimensions=[1 1 1]  BrickDimensionUnits=m  CylinderRadius=1  CylinderRadiusUnits=m  CylinderLength=1  CylinderLengthUnits=m  SphereRadius=1  SphereRadiusUnits=m  EllipsoidRadii=[1 1 1]  EllipsoidRadiiUnits=m  ExtrusionCrossSection=[1 1; -1 1; -1 -1; 1 -1]  ExtrusionCrossSectionUnits=m  ExtrusionLength=1  ExtrusionLengthUnits=m  PolygonNumSides=3  PolygonOuterRadius=1  PolygonOuterRadiusUnits=m  ExtGeomFileType=STL  ExtGeomFileName=.\geometry\wec4_reactor.stl  ExtGeomFileUnits=m  RevolutionCrossSection=[1 1; 1 -1; 2 -1; 2 1]  RevolutionCrossSectionUnits=m  RevolutionExtent=Full  RevolutionAngle=180  RevolutionAngleUnits=deg
  External Force and Torque : sm_lib/Forces and Torques/External Force and Torque  ForceResolutionFrame=World  EnableForceX=off  EnableForceY=off  EnableForceZ=off  EnableForce=on  TorqueResolutionFrame=World  EnableTorqueX=off  EnableTorqueY=off  EnableTorqueZ=off  EnableTorque=on
  Motion Sensor : Subsystem
  Rigid Transform (Setup CG) : sm_lib/Frames and Transforms/Rigid Transform  TranslationMethod=Cartesian  TranslationStandardOffset=0  TranslationLengthUnit=m  TranslationStandardAxis=+Z  TranslationCartesianOffset=body.cg  TranslationROffset=0  TranslationROffsetUnits=m  TranslationZOffset=0  TranslationZOffsetUnits=m  TranslationThetaOffset=0  TranslationThetaOffsetUnits=deg  RotationMethod=None  RotationAngleUnits=rad  RotationStandardAxis=+Y  RotationAngle=0.05  RotationArbitraryAxis=[0.57735026918962584 0.57735026918962584 0.57735026918962584]  FollAlignAxisA=+X  BaseAlignAxisA=+Y  FollAlignAxisB=+Y  BaseAlignAxisB=+Z  RotationSequenceAxes=FollowerAxes  RotationSequence=XYX  RotationSequenceAngles=[0 0 0]  RotationSequenceAnglesUnits=deg  RotationMatrix=[1 0 0; 0 1 0; 0 0 1]
  Rigid Transform (Setup Initial Disp) : sm_lib/Frames and Transforms/Rigid Transform  TranslationMethod=Cartesian  TranslationStandardOffset=0  TranslationLengthUnit=m  TranslationStandardAxis=+Z  TranslationCartesianOffset=body.initDisp.initLinDisp  TranslationROffset=0  TranslationROffsetUnits=m  TranslationZOffset=0  TranslationZOffsetUnits=m  TranslationThetaOffset=0  TranslationThetaOffsetUnits=deg  RotationMethod=ArbitraryAxis  RotationAngleUnits=rad  RotationStandardAxis=+Y  RotationAngle=body.initDisp.initAngularDispAngle  RotationArbitraryAxis=body.initDisp.initAngularDispAxis  FollAlignAxisA=+X  BaseAlignAxisA=+Y  FollAlignAxisB=+Y  BaseAlignAxisB=+Z  RotationSequenceAxes=FollowerAxes  RotationSequence=XYX  RotationSequenceAngles=[0 0 0]  RotationSequenceAnglesUnits=deg  RotationMatrix=[1 0 0; 0 1 0; 0 0 1]
  Selector : Selector  InputPortWidth=6  IndexOptions=Index vector (dialog)  Indices=[1:3]  OutputSizes=1
  Selector1 : Selector  InputPortWidth=6  IndexOptions=Index vector (dialog)  Indices=[4:6]  OutputSizes=1
  Simulink-PS Converter1 : nesl_utility/Simulink-PS Converter  PhysicalDomain=network_engine_domain  SubClassName=ps_input  LeftPortType=input  RightPortType=output  PseudoPeriodic=off  Frequencies=[]  NoiseDistribution=none  NoiseParameters=[]  Unit=1  AffineConversion=off  InputFiltering=off  SimscapeFilterOrder=1  InputFilterTimeConstant=0.001  UdotUserProvided=1
  Simulink-PS Converter2 : nesl_utility/Simulink-PS Converter  PhysicalDomain=network_engine_domain  SubClassName=ps_input  LeftPortType=input  RightPortType=output  PseudoPeriodic=off  Frequencies=[]  NoiseDistribution=none  NoiseParameters=[]  Unit=1  AffineConversion=off  InputFiltering=off  SimscapeFilterOrder=1  InputFilterTimeConstant=0.001  UdotUserProvided=1
  World Frame : sm_lib/Frames and Transforms/World Frame
  Conn Free Surface : PMIOPort  Port=1  Side=Right
  Response : Outport
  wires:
  Total Force/1 -> Selector1/1, Selector/1
  Selector/1 -> Simulink-PS Converter1/1
  Selector1/1 -> Simulink-PS Converter2/1
  Motion Sensor/1(Response) -> Response/1
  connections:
  External Force and Torque/LConn1 -- Simulink-PS Converter1/RConn1
  External Force and Torque/LConn2 -- Simulink-PS Converter2/RConn1
  Rigid Transform (Setup Initial Disp)/RConn1 -- Body Properties/RConn1 -- External Force and Torque/RConn1 -- Motion Sensor/RConn1
  Conn Free Surface/RConn1 -- Rigid Transform (Setup CG)/LConn1
  Rigid Transform (Setup Initial Disp)/LConn1 -- Rigid Transform (Setup CG)/RConn1
  World Frame/RConn1 -- Motion Sensor/LConn1

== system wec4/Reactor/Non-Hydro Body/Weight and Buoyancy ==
  Add1 : Sum  Inputs=+-
  Assignment (Add Net Bouyancy Force to Z-Direction) : Assignment  IndexOptions=Index vector (dialog)  Indices=3  OutputSizes=1
  Body Mass : Constant  Value=body.mass
  Constant1 : Constant  Value=[0 0 0 0 0 0]
  Gravity : Constant  Value=simu.g
  Product : Product
  Product1 : Product  Inputs=3
  Volume : Constant  Value=body.dispVol
  Water Density : Constant  Value=simu.rho
  Out1 : Outport
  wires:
  Add1/1 -> Assignment (Add Net Bouyancy Force to Z-Direction)/2
  Product1/1 -> Add1/2  "F_Buoyancy"
  Product/1 -> Add1/1  "F_Gravity"
  Water Density/1 -> Product1/1  "rho"
  Gravity/1 -> Product/1, Product1/2  "g"
  Volume/1 -> Product1/3  "Vol"
  Assignment (Add Net Bouyancy Force to Z-Direction)/1 -> Out1/1  "F_Restoring"
  Constant1/1 -> Assignment (Add Net Bouyancy Force to Z-Direction)/1
  Body Mass/1 -> Product/2  "m"

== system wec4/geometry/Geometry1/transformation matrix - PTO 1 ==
  PsiS : Inport
  rXs : Inport  Port=2
  rYs : Inport  Port=3
  PsiF : Inport  Port=4
  rXf : Inport  Port=5
  rYf : Inport  Port=6
  rZs : Inport  Port=7
  rZf : Inport  Port=8
  thetaS : Inport  Port=9
  thetaF : Inport  Port=10
  PhiF : Inport  Port=11
  PhiS : Inport  Port=12
  x_s : Inport  Port=13
  x_f : Inport  Port=14
  y_s : Inport  Port=15
  y_f : Inport  Port=16
  z_s : Inport  Port=17
  z_f : Inport  Port=18
  Abs : Abs
  Abs1 : Abs
  Abs2 : Abs
  Constant : Constant  Value=abs(rCogSpar-rCogFloater)
  Sum12 : Sum  Inputs=+-
  Sum13 : Sum  Inputs=++-
  Sum14 : Sum  Inputs=+-
  Sum15 : Sum  Inputs=++-
  Sum16 : Sum  Inputs=--
  Sum17 : Sum  Inputs=-++
  Sum18 : Sum  Inputs=|++
  pitch Spar : Subsystem
  pitch floater : Subsystem
  roll Spar : Subsystem
  roll floater : Subsystem
  yaw Floater : Subsystem
  yaw Spar : Subsystem
  zeta : Outport
  mu : Outport  Port=2
  eta : Outport  Port=3
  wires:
  Sum18/1 -> Abs/1
  Sum15/1 -> Abs1/1
  Sum13/1 -> Abs2/1
  Constant/1 -> Sum18/2
  Sum17/1 -> Sum18/1
  z_f/1 -> Sum17/3
  z_s/1 -> Sum17/1
  Sum16/1 -> Sum17/2
  y_f/1 -> Sum15/3
  y_s/1 -> Sum15/1
  Sum14/1 -> Sum15/2
  roll Spar/1(d_ys_theta) -> Sum14/1
  x_f/1 -> Sum13/3
  x_s/1 -> Sum13/1
  Sum12/1 -> Sum13/2
  Abs/1 -> eta/1
  Abs1/1 -> mu/1
  Abs2/1 -> zeta/1
  rXs/1 -> yaw Spar/1(Xs)
  PsiS/1 -> yaw Spar/2(PsiS)
  rYs/1 -> yaw Spar/3(Ys)
  yaw Spar/2(d_ys_psi) -> roll Spar/1(y_s)
  thetaS/1 -> roll Spar/2(theta)
  rZs/1 -> pitch Spar/3(Zs)
  yaw Spar/1(d_xs_psi) -> pitch Spar/1(Xs)
  PhiS/1 -> pitch Spar/2(Phi)
  roll Spar/2(d_zs_theta) -> Sum16/1
  pitch Spar/1(d_xs_phi) -> Sum12/1
  pitch Spar/2(d_zs_phi) -> roll Spar/3(z_s)
  rXf/1 -> yaw Floater/1(x_f)
  PsiF/1 -> yaw Floater/2(psiF)
  rYf/1 -> yaw Floater/3(y_f)
  yaw Floater/2(d_yf_psi) -> roll floater/1(y_f)
  thetaF/1 -> roll floater/2(thetaF)
  rZf/1 -> pitch floater/3(z_f)
  roll floater/1(d_yf_theta) -> Sum14/2
  yaw Floater/1(d_xf_psi) -> pitch floater/1(x_f)
  PhiF/1 -> pitch floater/2(phiF)
  roll floater/2(d_zf_theta) -> Sum16/2
  pitch floater/1(d_xf_phi) -> Sum12/2
  pitch floater/2(d_zf_phi) -> roll floater/3(z_f)

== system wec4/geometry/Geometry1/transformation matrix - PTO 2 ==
  PsiS : Inport
  rXs : Inport  Port=2
  rYs : Inport  Port=3
  PsiF : Inport  Port=4
  rXf : Inport  Port=5
  rYf : Inport  Port=6
  rZs : Inport  Port=7
  rZf : Inport  Port=8
  thetaS : Inport  Port=9
  thetaF : Inport  Port=10
  PhiF : Inport  Port=11
  PhiS : Inport  Port=12
  x_s : Inport  Port=13
  x_f : Inport  Port=14
  y_s : Inport  Port=15
  y_f : Inport  Port=16
  z_s : Inport  Port=17
  z_f : Inport  Port=18
  Abs : Abs
  Abs1 : Abs
  Abs2 : Abs
  Constant : Constant  Value=abs(rCogSpar-rCogFloater)
  Sum12 : Sum  Inputs=+-
  Sum13 : Sum  Inputs=++-
  Sum14 : Sum  Inputs=+-
  Sum15 : Sum  Inputs=++-
  Sum16 : Sum  Inputs=--
  Sum17 : Sum  Inputs=-++
  Sum18 : Sum  Inputs=|++
  pitch Spar : Subsystem
  pitch floater : Subsystem
  roll Spar : Subsystem
  roll floater : Subsystem
  yaw Floater : Subsystem
  yaw Spar : Subsystem
  zeta : Outport
  mu : Outport  Port=2
  eta : Outport  Port=3
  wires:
  pitch floater/2(d_zf_phi) -> roll floater/3(z_f)
  pitch floater/1(d_xf_phi) -> Sum12/2
  roll floater/2(d_zf_theta) -> Sum16/2
  PhiF/1 -> pitch floater/2(phiF)
  yaw Floater/1(d_xf_psi) -> pitch floater/1(x_f)
  roll floater/1(d_yf_theta) -> Sum14/2
  rZf/1 -> pitch floater/3(z_f)
  thetaF/1 -> roll floater/2(thetaF)
  yaw Floater/2(d_yf_psi) -> roll floater/1(y_f)
  rYf/1 -> yaw Floater/3(y_f)
  PsiF/1 -> yaw Floater/2(psiF)
  rXf/1 -> yaw Floater/1(x_f)
  pitch Spar/2(d_zs_phi) -> roll Spar/3(z_s)
  pitch Spar/1(d_xs_phi) -> Sum12/1
  roll Spar/2(d_zs_theta) -> Sum16/1
  PhiS/1 -> pitch Spar/2(Phi)
  yaw Spar/1(d_xs_psi) -> pitch Spar/1(Xs)
  rZs/1 -> pitch Spar/3(Zs)
  thetaS/1 -> roll Spar/2(theta)
  yaw Spar/2(d_ys_psi) -> roll Spar/1(y_s)
  rYs/1 -> yaw Spar/3(Ys)
  PsiS/1 -> yaw Spar/2(PsiS)
  rXs/1 -> yaw Spar/1(Xs)
  Abs2/1 -> zeta/1
  Abs1/1 -> mu/1
  Abs/1 -> eta/1
  Sum12/1 -> Sum13/2
  x_s/1 -> Sum13/1
  x_f/1 -> Sum13/3
  roll Spar/1(d_ys_theta) -> Sum14/1
  Sum14/1 -> Sum15/2
  y_s/1 -> Sum15/1
  y_f/1 -> Sum15/3
  Sum16/1 -> Sum17/2
  z_s/1 -> Sum17/1
  z_f/1 -> Sum17/3
  Sum17/1 -> Sum18/1
  Constant/1 -> Sum18/2
  Sum13/1 -> Abs2/1
  Sum15/1 -> Abs1/1
  Sum18/1 -> Abs/1

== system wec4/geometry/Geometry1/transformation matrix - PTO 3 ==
  PsiS : Inport
  rXs : Inport  Port=2
  rYs : Inport  Port=3
  PsiF : Inport  Port=4
  rXf : Inport  Port=5
  rYf : Inport  Port=6
  rZs : Inport  Port=7
  rZf : Inport  Port=8
  thetaS : Inport  Port=9
  thetaF : Inport  Port=10
  PhiF : Inport  Port=11
  PhiS : Inport  Port=12
  x_s : Inport  Port=13
  x_f : Inport  Port=14
  y_s : Inport  Port=15
  y_f : Inport  Port=16
  z_s : Inport  Port=17
  z_f : Inport  Port=18
  Abs : Abs
  Abs1 : Abs
  Abs2 : Abs
  Constant : Constant  Value=abs(rCogSpar-rCogFloater)
  Sum12 : Sum  Inputs=+-
  Sum13 : Sum  Inputs=++-
  Sum14 : Sum  Inputs=+-
  Sum15 : Sum  Inputs=++-
  Sum16 : Sum  Inputs=--
  Sum17 : Sum  Inputs=-++
  Sum18 : Sum  Inputs=|++
  pitch Spar : Subsystem
  pitch floater : Subsystem
  roll Spar : Subsystem
  roll floater : Subsystem
  yaw Floater : Subsystem
  yaw Spar : Subsystem
  zeta : Outport
  mu : Outport  Port=2
  eta : Outport  Port=3
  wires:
  pitch floater/2(d_zf_phi) -> roll floater/3(z_f)
  pitch floater/1(d_xf_phi) -> Sum12/2
  roll floater/2(d_zf_theta) -> Sum16/2
  PhiF/1 -> pitch floater/2(phiF)
  yaw Floater/1(d_xf_psi) -> pitch floater/1(x_f)
  roll floater/1(d_yf_theta) -> Sum14/2
  rZf/1 -> pitch floater/3(z_f)
  thetaF/1 -> roll floater/2(thetaF)
  yaw Floater/2(d_yf_psi) -> roll floater/1(y_f)
  rYf/1 -> yaw Floater/3(y_f)
  PsiF/1 -> yaw Floater/2(psiF)
  rXf/1 -> yaw Floater/1(x_f)
  pitch Spar/2(d_zs_phi) -> roll Spar/3(z_s)
  pitch Spar/1(d_xs_phi) -> Sum12/1
  roll Spar/2(d_zs_theta) -> Sum16/1
  PhiS/1 -> pitch Spar/2(Phi)
  yaw Spar/1(d_xs_psi) -> pitch Spar/1(Xs)
  rZs/1 -> pitch Spar/3(Zs)
  thetaS/1 -> roll Spar/2(theta)
  yaw Spar/2(d_ys_psi) -> roll Spar/1(y_s)
  rYs/1 -> yaw Spar/3(Ys)
  PsiS/1 -> yaw Spar/2(PsiS)
  rXs/1 -> yaw Spar/1(Xs)
  Abs2/1 -> zeta/1
  Abs1/1 -> mu/1
  Abs/1 -> eta/1
  Sum12/1 -> Sum13/2
  x_s/1 -> Sum13/1
  x_f/1 -> Sum13/3
  roll Spar/1(d_ys_theta) -> Sum14/1
  Sum14/1 -> Sum15/2
  y_s/1 -> Sum15/1
  y_f/1 -> Sum15/3
  Sum16/1 -> Sum17/2
  z_s/1 -> Sum17/1
  z_f/1 -> Sum17/3
  Sum17/1 -> Sum18/1
  Constant/1 -> Sum18/2
  Sum13/1 -> Abs2/1
  Sum15/1 -> Abs1/1
  Sum18/1 -> Abs/1

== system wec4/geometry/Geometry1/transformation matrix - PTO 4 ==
  PsiS : Inport
  rXs : Inport  Port=2
  rYs : Inport  Port=3
  PsiF : Inport  Port=4
  rXf : Inport  Port=5
  rYf : Inport  Port=6
  rZs : Inport  Port=7
  rZf : Inport  Port=8
  thetaS : Inport  Port=9
  thetaF : Inport  Port=10
  PhiF : Inport  Port=11
  PhiS : Inport  Port=12
  x_s : Inport  Port=13
  x_f : Inport  Port=14
  y_s : Inport  Port=15
  y_f : Inport  Port=16
  z_s : Inport  Port=17
  z_f : Inport  Port=18
  Abs : Abs
  Abs1 : Abs
  Abs2 : Abs
  Constant : Constant  Value=abs(rCogSpar-rCogFloater)
  Sum12 : Sum  Inputs=+-
  Sum13 : Sum  Inputs=++-
  Sum14 : Sum  Inputs=+-
  Sum15 : Sum  Inputs=++-
  Sum16 : Sum  Inputs=--
  Sum17 : Sum  Inputs=-++
  Sum18 : Sum  Inputs=|++
  pitch Spar : Subsystem
  pitch floater : Subsystem
  roll Spar : Subsystem
  roll floater : Subsystem
  yaw Floater : Subsystem
  yaw Spar : Subsystem
  zeta : Outport
  mu : Outport  Port=2
  eta : Outport  Port=3
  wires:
  pitch floater/2(d_zf_phi) -> roll floater/3(z_f)
  pitch floater/1(d_xf_phi) -> Sum12/2
  roll floater/2(d_zf_theta) -> Sum16/2
  PhiF/1 -> pitch floater/2(phiF)
  yaw Floater/1(d_xf_psi) -> pitch floater/1(x_f)
  roll floater/1(d_yf_theta) -> Sum14/2
  rZf/1 -> pitch floater/3(z_f)
  thetaF/1 -> roll floater/2(thetaF)
  yaw Floater/2(d_yf_psi) -> roll floater/1(y_f)
  rYf/1 -> yaw Floater/3(y_f)
  PsiF/1 -> yaw Floater/2(psiF)
  rXf/1 -> yaw Floater/1(x_f)
  pitch Spar/2(d_zs_phi) -> roll Spar/3(z_s)
  pitch Spar/1(d_xs_phi) -> Sum12/1
  roll Spar/2(d_zs_theta) -> Sum16/1
  PhiS/1 -> pitch Spar/2(Phi)
  yaw Spar/1(d_xs_psi) -> pitch Spar/1(Xs)
  rZs/1 -> pitch Spar/3(Zs)
  thetaS/1 -> roll Spar/2(theta)
  yaw Spar/2(d_ys_psi) -> roll Spar/1(y_s)
  rYs/1 -> yaw Spar/3(Ys)
  PsiS/1 -> yaw Spar/2(PsiS)
  rXs/1 -> yaw Spar/1(Xs)
  Abs2/1 -> zeta/1
  Abs1/1 -> mu/1
  Abs/1 -> eta/1
  Sum12/1 -> Sum13/2
  x_s/1 -> Sum13/1
  x_f/1 -> Sum13/3
  roll Spar/1(d_ys_theta) -> Sum14/1
  Sum14/1 -> Sum15/2
  y_s/1 -> Sum15/1
  y_f/1 -> Sum15/3
  Sum16/1 -> Sum17/2
  z_s/1 -> Sum17/1
  z_f/1 -> Sum17/3
  Sum17/1 -> Sum18/1
  Constant/1 -> Sum18/2
  Sum13/1 -> Abs2/1
  Sum15/1 -> Abs1/1
  Sum18/1 -> Abs/1

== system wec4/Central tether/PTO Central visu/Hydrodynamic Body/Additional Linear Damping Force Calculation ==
  Velocity : Inport
  Additional Linear Damping Matrix (diagonal) : Constant  Value=body.hydroForce.linearDamping
  Product1 : Product  Multiplication=Matrix(*)
  F_LinearDamping : Outport
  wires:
  Velocity/1 -> Product1/2  "v"
  Product1/1 -> F_LinearDamping/1  "F_LinearDamping"
  Additional Linear Damping Matrix (diagonal)/1 -> Product1/1  "C"
